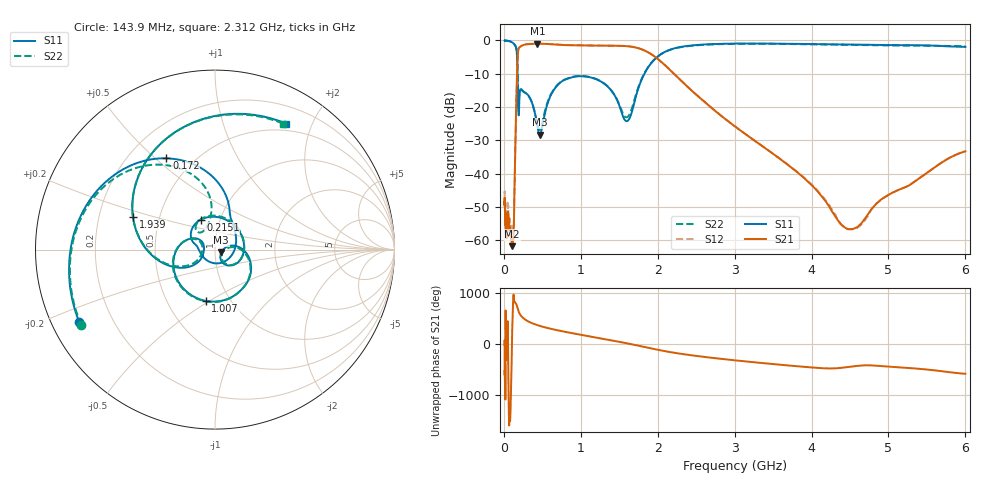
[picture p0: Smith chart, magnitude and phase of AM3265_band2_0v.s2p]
!Agilent Technologies,E8364B,MY43040894,A.07.50.67
!Agilent E8364B: A.07.50.67
!Date: Friday, May 09, 2025 07:21:52
!Correction: S11(Full 2 Port(1,2))
!S21(Full 2 Port(1,2))
!S12(Full 2 Port(1,2))
!S22(Full 2 Port(1,2))
!S2P File: Measurements: S11, S21, S12, S22:Log Frequency Sweep
# Hz S  dB  R 50
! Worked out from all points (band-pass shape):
!   3201 points, 10 MHz to 6 GHz, reference 50 ohm
!   highest |S21| = -0.95 dB at 436.5 MHz (marker M1); lowest = -61.9 dB at 107.3 MHz (marker M2)
!   |S21| within 3 dB of the highest: 183.1 MHz to 1.905 GHz (1.721 GHz wide, 165 % of centre)
!   lowest |S11| = -28.3 dB at 467.2 MHz (marker M3), VSWR 1.08, Z = 53.6 - j1.72 ohm
!   |S11| at or under -10 dB: 178.9 MHz to 1.827 GHz (1.648 GHz wide, 164 % of centre)
!   |S22| runs from -26.9 to 0.0 dB; largest |S21 - S12| = 0.0094
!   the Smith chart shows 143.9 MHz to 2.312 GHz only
!   S11 on the Smith chart (normalised r, x): 143.9 MHz: 0.08, -0.25; 172 MHz: 0.36, +0.54; 215.1 MHz: 0.81, +0.28; 1.007 GHz: 0.77, -0.48; 1.939 GHz: 0.35, +0.17; 2.312 GHz: 0.41, +1.63
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1e7  -0.03 -7.8  -49.26 -24.4  -50.00 92.5  -0.06 -8.0
2.908064e7  -0.04 -22.5  -58.46 -134.0  -55.72 128.8  -0.04 -22.5
8.439949e7  -0.27 -70.6  -58.00 -6.4  -56.38 -154.7  -0.31 -70.8
1.072804e8  -0.55 -95.9  -61.85 163.7  -57.41 150.8  -0.56 -95.7
1.439268e8  -1.34 -152.0  -36.96 96.5  -36.85 95.7  -1.36 -150.6
1.719528e8  -4.79 118.0  -9.72 13.2  -9.67 13.3  -4.63 126.4
2.15102e8  -14.67 115.8  -1.85 -154.0  -1.81 -154.0  -14.43 105.5
2.44949e8  -15.25 51.5  -1.44 154.3  -1.41 154.3  -15.12 47.4
4.364931e8  -25.92 -54.1  -0.95 5.4  -0.93 5.4  -25.27 -48.7
4.671919e8  -28.34 -24.8  -0.97 -9.1  -0.93 -9.1  -26.91 -23.1
7.123273e8  -13.12 -24.7  -1.26 -99.8  -1.22 -99.8  -12.98 -28.2
1.006638e9  -10.75 -100.1  -1.49 175.3  -1.47 175.3  -10.67 -102.4
1.310606e9  -13.07 -175.4  -1.54 92.8  -1.51 92.8  -13.01 -175.9
1.591054e9  -24.26 174.4  -1.69 12.9  -1.67 12.9  -23.09 176.2
1.939251e9  -6.17 158.5  -4.48 -98.0  -4.46 -98.0  -6.13 157.9
2.067357e9  -3.76 121.3  -6.85 -136.5  -6.83 -136.4  -3.77 121.5
2.312241e9  -1.88 60.7  -12.29 162.0  -12.26 162.0  -1.96 61.6
3.202913e9  -0.90 -91.5  -29.19 6.1  -29.18 5.9  -0.98 -91.5
3.818953e9  -1.02 -178.2  -39.71 -80.3  -39.58 -80.0  -1.08 -179.7
4.490206e9  -1.21 91.9  -56.74 -91.7  -56.74 -92.8  -1.31 90.5
5.185309e9  -1.41 1.1  -44.44 -107.6  -44.43 -107.3  -1.52 1.3
6e9  -1.93 -96.9  -33.34 132.3  -33.30 132.4  -1.68 -96.5
